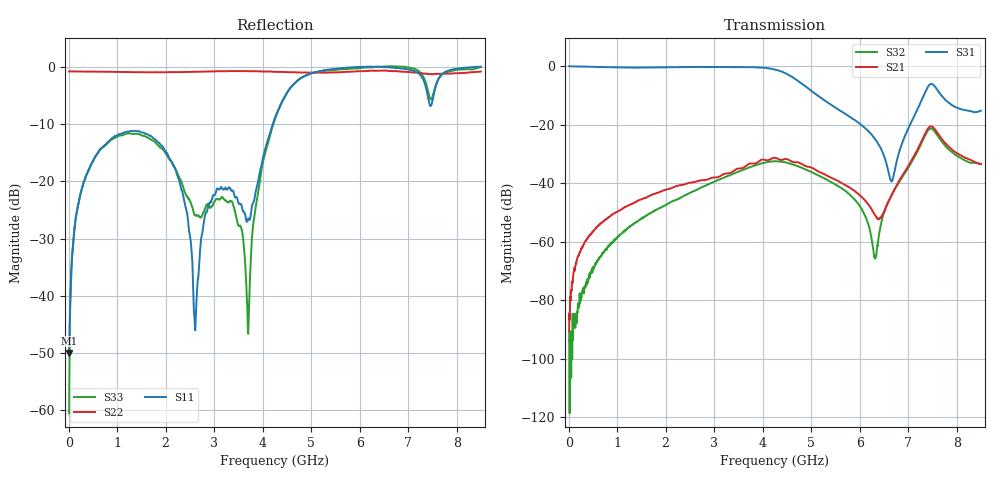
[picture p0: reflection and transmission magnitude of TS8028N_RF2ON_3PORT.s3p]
!Created with skrf (http://scikit-rf.org).
# GHz S RI R 50.0
!freq ReS11 ImS11 ReS12 ImS12 ReS13 ImS13
! ReS21 ImS21 ReS22 ImS22 ReS23 ImS23
! ReS31 ImS31 ReS32 ImS32 ReS33 ImS33
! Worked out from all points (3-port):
!   1601 points, 10 MHz to 8.5 GHz, reference 50 ohm
!   strongest paths, dB at 10 MHz, 2.132 GHz, 4.255 GHz, 6.378 GHz, 8.5 GHz:
!     S31: 0.0, -0.4, -1.2, -26.4, -15.2
!     S21: -90.4, -41.6, -31.4, -52.2, -33.5
!     S32: -90.8, -46.3, -32.5, -60.1, -33.5
!   lowest |S11| = -50.0 dB at 10 MHz (marker M1), VSWR 1.01, Z = 50.3 + j0.0306 ohm
!   |S11| at or under -10 dB: start of sweep to 4.21 GHz
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0.01  0.00314 0.000305  1.4e-05 1.1e-05  0.9945 -0.0096
      -2.82e-05 1.05e-05  -0.9134 0.00502  -7.89e-06 -1.51e-05
      0.9944 -0.00962  5.37e-06 -2.84e-05  0.000628 0.000698
0.6520563  -0.0599 -0.1805  -0.000259 0.002  0.9088 -0.3127
           -0.000255 0.002  -0.8883 0.1845  -0.000549 2.45e-05
           0.9089 -0.3124  -0.000554 2.41e-05  -0.0523 -0.1815
2.015763  -0.1142 -0.1379  -6.26e-05 0.00777  0.5422 -0.7874
          -2.75e-05 0.00779  -0.7333 0.519  -0.00304 0.003
          0.5415 -0.7876  -0.00305 0.00301  -0.1396 -0.0992
2.610063  -0.00441 0.00231  0.00127 0.0105  0.2534 -0.9317
          0.00123 0.0105  -0.6231 0.6572  -0.00381 0.00639
          0.2533 -0.9312  -0.00377 0.00643  -0.00999 -0.0498
3.697844  0.0135 0.0447  0.00604 0.0199  -0.4562 -0.8411
          0.00599 0.0199  -0.4174 0.8165  0.00315 0.0179
          -0.4563 -0.8409  0.00316 0.0179  -0.00213 -0.00427
4.255  -0.1516 0.3272  0.0204 0.0179  -0.785 -0.3844
       0.0204 0.0178  -0.2952 0.8574  0.0179 0.0153
       -0.7846 -0.383  0.018 0.0154  -0.0842 0.3388
6.319131  0.2947 0.9607  0.00247 0.00132  -0.0502 0.0264
          0.00249 0.00131  0.2434 0.892  0.000343 0.000349
          -0.0502 0.0265  0.000347 0.000382  0.7962 0.6024
6.669344  0.3397 0.9238  -0.0031 0.00561  -0.00553 -0.00931
          -0.00306 0.00566  0.2904 0.872  -0.00357 0.00536
          -0.00558 -0.00932  -0.00361 0.00534  0.8018 0.6179
7.428138  0.1734 0.467  0.0273 0.0851  -0.1027 -0.4548
          0.0274 0.085  0.4302 0.75  0.0439 0.0698
          -0.1034 -0.4548  0.0438 0.07  0.4477 0.3537
8.5  -0.4366 0.9042  0.0207 -0.00419  -0.1728 0.00373
     0.0207 -0.00417  0.6777 0.6072  0.0164 -0.013
     -0.1728 0.0037  0.0165 -0.013  0.3666 0.9251
